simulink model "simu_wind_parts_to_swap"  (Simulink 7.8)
settings: Solver=ode45  StartTime=0.0  StopTime=10.0  RelTol=1e-3
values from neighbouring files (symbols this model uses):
  a = 14.2e-3/2    (= 0.0071)    [hybrid_wind.m]    (also in measurements.m)
  an = modal_coeff(:,1)    [hybrid_wind.m]
  c = 344    [hybrid_wind.m]    (also in measurements.m)
  fs = 1/Ts    (= 40000)    [hybrid_wind.m]    (also in measurements.m)
  mu_s = 0.8    [bowed_string_hyperbolic.m]
  PM = 50    [bowed_string_hyperbolic.m]    (also in lip_reed.m = 20; single_reed.m = 100)
  Qn = modal_coeff(:,3)    [hybrid_wind.m]
  rho = 1.204    [hybrid_wind.m]    (also in measurements.m)
  St = a^2 *pi    (= 0.000158367685667)    [hybrid_wind.m]    (also in measurements.m)
  Ts = 25e-6    (= 2.5e-05)    [hybrid_wind.m]    (also in measurements.m)
  wn = modal_coeff(:,2)    [hybrid_wind.m]
  wr_vect = [timevect_sigs'  wr_start+ (sawtooth(timevect_sigs/5*2*pi)+1)'/2*(wr_stop-wr_start) ]    [lip_reed.m]
undefined symbols (not defined in the file or in its folder): Bl, cell2mat, d1, d2, dL, He_d, Lt, Mms, modal_coeff, n1, Qts, Re, Sd, w_rms, wLS, ws, Zcstring, zetaLS
libraries: fl_lib x7, simulink x5, nesl_utility x4

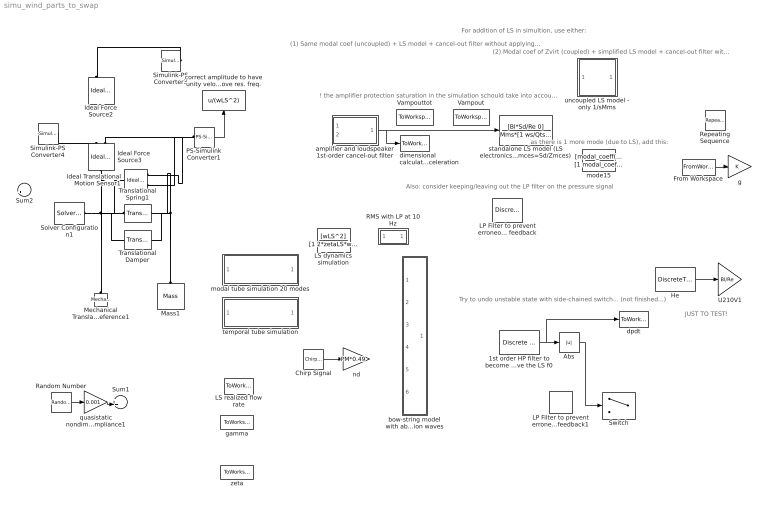
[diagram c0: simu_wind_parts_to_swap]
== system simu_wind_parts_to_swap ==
  note: For addition of LS in simultion, use either:
  note: (1) Same modal coef (uncoupled) + LS model + cancel-out filter without applying the FB
  note: (2) Modal coef of Zvirt (coupled) + simplified LS model + cancel-out filter with applying the FB
  note: as there is 1 more mode (due to LS), add this:
  note: Also: consider keeping/leaving out the LP filter on the pressure signal
  note: Try to undo unstable state with side-chained switch... (not finished...)
  note: ! the amplifier protection saturation in the simulation schould take into account the uncoupling feedback signal...
  note: JUST TO TEST!
  1st order HP filter to become a flat  amp and 0 phase flow rate response above the LS f0 : simulink/Discrete/Discrete Derivative  gainval=1.0  ICPrevScaledInput=0.0  InputProcessing=Inherited  OutMin=[]  OutMax=[]  OutDataType=fixdt(1, 16)  OutScaling=2^-10  DoSatur=off
  Abs : Abs
  Chirp Signal : simulink/Sources/Chirp Signal  f1=0.1  T=5  f2=1000
  From Workspace : FromWorkspace  VariableName=sample  SampleTime=0
  He : DiscreteTransferFcn  Numerator=cell2mat(He_d.num)  Denominator=cell2mat(He_d.den)  SampleTime=Ts
  Ideal Force Source2 : fl_lib/Mechanical/Mechanical Sources/Ideal Force Source  v_Log=off  f_Log=off  LocalVarNames=|v|f  LocalVarDescs=|v|f  LocalVarLogging=[0 0]
  Ideal Force Source3 : fl_lib/Mechanical/Mechanical Sources/Ideal Force Source  v_Log=off  f_Log=off  LocalVarNames=|v|f  LocalVarDescs=|v|f  LocalVarLogging=[0 0]
  Ideal Translational Motion Sensor1 : fl_lib/Mechanical/Mechanical Sensors/Ideal Translational Motion Sensor  offset=0 m  v_Log=off  f_Log=off  x_Log=off  LocalVarNames=|v|f|x  LocalVarDescs=|v|f|x  LocalVarLogging=[0 0 0]
  LP Filter to prevent erroneous high freq feedback : DiscreteFilter  Numerator=HdLP.ScaleValues(1)*HdLP.sosMatrix(1:end/2)  Denominator=HdLP.ScaleValues(2)*HdLP.sosMatrix(1+end/2:end)  SampleTime=Ts
  LP Filter to prevent erroneous high freq feedback1 : DiscreteFilter  Numerator=HdLP.ScaleValues(1)*HdLP.sosMatrix(1:end/2)  Denominator=HdLP.ScaleValues(2)*HdLP.sosMatrix(1+end/2:end)  SampleTime=Ts
  LS dynamics simulation : TransferFcn  Numerator=[wLS^2]  Denominator=[1 2*zetaLS*wLS wLS^2]
  LS realized flow rate : ToWorkspace  VariableName=U_LS  SampleTime=-1  SaveFormat=Structure
  Mass1 : fl_lib/Mechanical/Translational Elements/Mass  mass=1/wLS^2 kg  initial_velocity=0 m/s  f_Log=off  LocalVarNames=|f  LocalVarDescs=|f  LocalVarLogging=0
  Mechanical Translational Reference1 : fl_lib/Mechanical/Translational Elements/Mechanical Translational Reference  f_Log=off  LocalVarNames=|f  LocalVarDescs=|f  LocalVarLogging=0
  PS-Simulink Converter1 : nesl_utility/PS-Simulink Converter  PhysicalDomain=network_engine_domain  LeftPortType=input  RightPortType=output  SubClassName=ps_output  Unit=1  AffineConversion=off
  RMS with LP at 10 Hz : Subsystem
  Random Number : RandomNumber  SampleTime=Ts
  Repeating Sequence : simulink/Sources/Repeating Sequence  rep_seq_t=wr_vect(:,1)/30  rep_seq_y=wr_vect(:,2)
  Simulink-PS Converter3 : nesl_utility/Simulink-PS Converter  PhysicalDomain=network_engine_domain  LeftPortType=input  RightPortType=output  SubClassName=ps_input  Unit=1  AffineConversion=off  InputFilterTimeConstant=.001  UdotUserProvided=0
  Simulink-PS Converter4 : nesl_utility/Simulink-PS Converter  PhysicalDomain=network_engine_domain  LeftPortType=input  RightPortType=output  SubClassName=ps_input  Unit=1  AffineConversion=off  InputFilterTimeConstant=.001  UdotUserProvided=0
  Solver Configuration1 : nesl_utility/Solver Configuration  PhysicalDomain=network_engine_domain  LeftPortType=input  RightPortType=generic  SubClassName=solver  DoDC=on  ResidualTolerance=1e-9  UseLocalSolver=on  LocalSolverChoice=NE_TRAPEZOIDAL_ADVANCER  LocalSolverSampleTime=1/fs  DoFixedCost=on  MaxNonlinIter=3  MaxModeIter=2  LinearAlgebra=Sparse  Accelerate=off  Profile=off  UseLocalSampling=off  DelaysMemoryBudget=1024
  Sum1 : Sum  Inputs=++|
  Sum2 : Sum  Inputs=|+-
  Switch : Switch  Threshold=50
  Translational Damper : fl_lib/Mechanical/Translational Elements/Translational Damper  D=2*zetaLS/wLS N/(m/s)  f_Log=off  v_Log=off  LocalVarNames=|f|v  LocalVarDescs=|f|v  LocalVarLogging=[0 0]
  Translational Spring1 : fl_lib/Mechanical/Translational Elements/Translational Spring  spr_rate=1 N/m  init_def=0 m  f_Log=off  v_Log=off  x_Log=off  LocalVarNames=|f|v|x  LocalVarDescs=|f|v|x  LocalVarLogging=[0 0 0]
  U210V1 : Gain  Gain=Bl/Re
  Vampout : ToWorkspace  VariableName=Vampout  SampleTime=-1  SaveFormat=Structure
  Vampouttot : ToWorkspace  VariableName=Vampouttot  SampleTime=-1  SaveFormat=Structure
  amplifier and loudspeaker 1st-order cancel-out filter : Subsystem
  bow-string model with absorbed torsion waves : Subsystem
  correct amplitude to have unity velocity above res. freq. : Fcn  Expr=u/(wLS^2)
  dimensional calculated flow acceleration : ToWorkspace  VariableName=A  SampleTime=-1  SaveFormat=Structure
  dpdt : ToWorkspace  VariableName=ddpdt  SampleTime=-1  SaveFormat=Structure
  g : Gain
  gamma : ToWorkspace  VariableName=gamma_vect_simu  SampleTime=-1  SaveFormat=Structure
  modal tube simulation 20 modes : Subsystem
  mode15 : TransferFcn  Numerator=[modal_coeff(15, 1) 0]  Denominator=[1 modal_coeff(15,2)/modal_coeff(15,3) modal_coeff(15,2)^2]
  nd : Gain  Gain=PM*0.49
  quasistatic nondimensional reed compliance1 : Gain  Gain=0.001
  standalone LS model (LS electronics&mechanics Bl*Sd/Re*Ymces=Sd/Zmces) : TransferFcn  Numerator=[Bl*Sd/Re 0]  Denominator=Mms*[1 ws/Qts (ws)^2]
  temporal tube simulation : Subsystem
  uncoupled LS model - only 1/sMms : Subsystem
  zeta : ToWorkspace  VariableName=zeta_vect_simu  SampleTime=-1  SaveFormat=Structure
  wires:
  PS-Simulink Converter1/1 -> correct amplitude to have unity velocity above res. freq./1
  correct amplitude to have unity velocity above res. freq./1 -> ?
  Chirp Signal/1 -> nd/1
  1st order HP filter to become a flat  amp and 0 phase flow rate response above the LS f0/1 -> Abs/1, dpdt/1
  Abs/1 -> Switch/2
  Random Number/1 -> quasistatic nondimensional reed compliance1/1
  ? -> Sum1/1  "p_nd"
  quasistatic nondimensional reed compliance1/1 -> Sum1/2
  amplifier and loudspeaker 1st-order cancel-out filter/1(V_amp_out) -> dimensional calculated flow acceleration/1, standalone LS model (LS electronics&mechanics Bl*Sd/Re*Ymces=Sd/Zmces)/1
  He/1 -> U210V1/1
  From Workspace/1 -> g/1
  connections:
  Simulink-PS Converter3/RConn1 -- Ideal Force Source2/RConn1
  Solver Configuration1/RConn1 -- Translational Damper/LConn1 -- Mechanical Translational Reference1/LConn1 -- Translational Spring1/LConn1 -- Ideal Translational Motion Sensor1/LConn1 -- Ideal Force Source3/LConn1
  Ideal Force Source3/RConn2 -- Ideal Translational Motion Sensor1/RConn1 -- Translational Spring1/RConn1 -- Translational Damper/RConn1 -- Mass1/LConn1
  Simulink-PS Converter4/RConn1 -- Ideal Force Source3/RConn1
  Ideal Translational Motion Sensor1/RConn3 -- PS-Simulink Converter1/LConn1

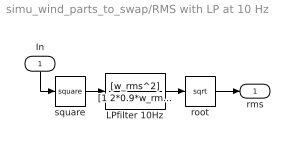
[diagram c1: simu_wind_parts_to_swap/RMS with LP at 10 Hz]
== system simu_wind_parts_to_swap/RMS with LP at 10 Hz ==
  In : Inport
  LPfilter 10Hz : TransferFcn  Numerator=[w_rms^2]  Denominator=[1 2*0.9*w_rms w_rms^2]
  root : Math  Operator=sqrt
  square : Math  Operator=square
  rms : Outport
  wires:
  square/1 -> LPfilter 10Hz/1
  LPfilter 10Hz/1 -> root/1
  In/1 -> square/1
  root/1 -> rms/1

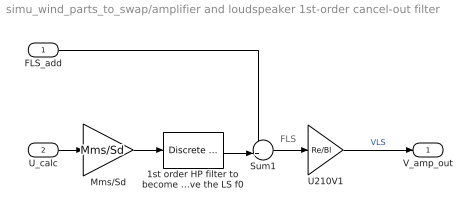
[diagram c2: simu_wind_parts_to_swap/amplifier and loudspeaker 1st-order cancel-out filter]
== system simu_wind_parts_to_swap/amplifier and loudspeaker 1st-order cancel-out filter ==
  note: FLS
  FLS_add : Inport
  U_calc : Inport  Port=2
  1st order HP filter to become a flat  amp and 0 phase flow rate response above the LS f0 : simulink/Discrete/Discrete Derivative  gainval=1.0  ICPrevScaledInput=0.0  InputProcessing=Inherited  OutMin=[]  OutMax=[]  OutDataType=fixdt(1, 16)  OutScaling=2^-10  DoSatur=off
  Mms/Sd : Gain  Gain=Mms/Sd
  Sum1 : Sum  Inputs=-+|
  U210V1 : Gain  Gain=Re/Bl
  V_amp_out : Outport
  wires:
  Sum1/1 -> U210V1/1
  Mms/Sd/1 -> 1st order HP filter to become a flat  amp and 0 phase flow rate response above the LS f0/1
  U210V1/1 -> V_amp_out/1  "VLS"
  U_calc/1 -> Mms/Sd/1
  1st order HP filter to become a flat  amp and 0 phase flow rate response above the LS f0/1 -> Sum1/2
  FLS_add/1 -> Sum1/1

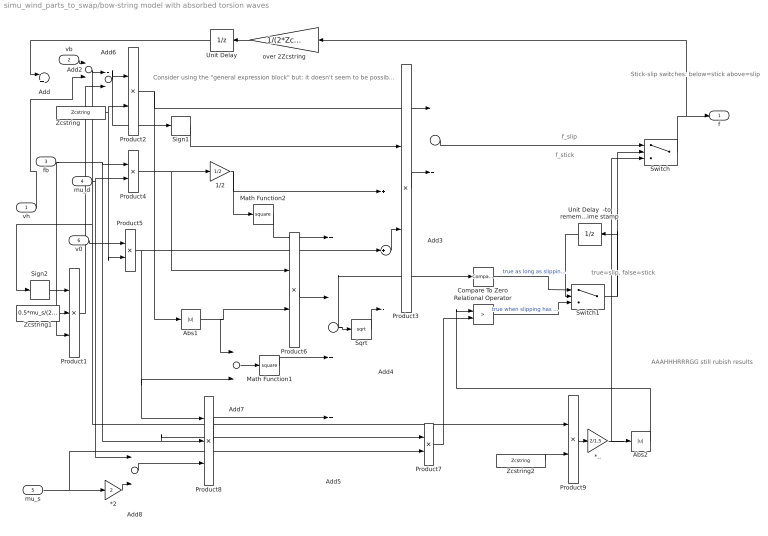
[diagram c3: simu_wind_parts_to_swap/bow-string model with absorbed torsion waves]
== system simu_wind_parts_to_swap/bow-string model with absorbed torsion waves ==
  note: Stick-slip switches: below=stick above=slip
  note: AAAHHHRRRGG still rubish results
  note: true=slip, false=stick
  note: f_stick
  note: f_slip
  note: Consider using the "general expression block" but: it doesn't seem to be possible to make it have more then 1 input! so this way may be more convenient if all parameters are provided as inputs...
  vh : Inport
  vb : Inport  Port=2
  fb : Inport  Port=3
  mu_d : Inport  Port=4
  mu_s : Inport  Port=5
  v0 : Inport  Port=6
  *.. : Gain  Gain=2/1.5
  *2 : Gain  Gain=2
  1/2 : Gain  Gain=1/2
  Abs1 : Abs
  Abs2 : Abs
  Add : Sum  Inputs=-+
  Add2 : Sum  Inputs=+-
  Add3 : Sum
  Add4 : Sum  Inputs=++-
  Add5 : Sum  Inputs=+-++
  Add6 : Sum  Inputs=+-
  Add7 : Sum
  Add8 : Sum  Inputs=+-
  Compare To Zero : simulink/Logic and Bit Operations/Compare To Zero  relop=>  OutDataTypeStr=uint8
  Math Function1 : Math  Operator=square
  Math Function2 : Math  Operator=square
  Product1 : Product  Inputs=3
  Product{2..7,9} (7 alike) : Product
  Product8 : Product  Inputs=3
  Relational Operator : RelationalOperator  Operator=>  OutDataTypeStr=boolean
  Sign1 : Signum
  Sign2 : Signum
  Sqrt : Sqrt
  Switch : Switch  Criteria=u2 > Threshold
  Switch1 : Switch  Criteria=u2 > Threshold
  Unit Delay : UnitDelay  SampleTime=-1
  Unit Delay  -to remember slip/stick state of previous time stamp : UnitDelay  SampleTime=-1
  Zcstring : Constant  Value=Zcstring
  Zcstring1 : Constant  Value=0.5*mu_s/(2*Zcstring)
  Zcstring2 : Constant  Value=Zcstring
  over 2Zcstring : Gain  Gain=1/(2*Zcstring)
  f : Outport
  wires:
  vb/1 -> Add2/1
  Zcstring/1 -> Product2/2, Product5/2
  Product2/1 -> Abs1/1, Add3/1
  Product3/1 -> Add3/2
  fb/1 -> Product4/1, Product8/2, Product7/1, Product1/3
  mu_d/1 -> Product4/2, Add8/1
  Product4/1 -> 1/2/1, Product6/1
  Product5/1 -> Add4/2, Add7/2, Product8/1
  v0/1 -> Product5/1
  Sqrt/1 -> Add4/3
  Sign1/1 -> Product3/1
  Add4/1 -> Product3/2
  Abs1/1 -> Product6/2, Add7/1
  1/2/1 -> Add4/1, Math Function2/1
  Add7/1 -> Math Function1/1
  mu_s/1 -> *2/1, Product7/2
  *2/1 -> Add8/2
  Add8/1 -> Product8/3
  Add5/1 -> Sqrt/1, Compare To Zero/1
  Math Function2/1 -> Add5/1
  Product6/1 -> Add5/2
  Math Function1/1 -> Add5/3
  Product8/1 -> Add5/4
  Add3/1 -> Switch/1
  Switch1/1 -> Unit Delay  -to remember slip/stick state of previous time stamp/1, Switch/2
  Product7/1 -> Relational Operator/2
  Switch/1 -> f/1, over 2Zcstring/1
  Unit Delay  -to remember slip/stick state of previous time stamp/1 -> Switch1/2
  over 2Zcstring/1 -> Unit Delay/1
  Compare To Zero/1 -> Switch1/1  "true as long as slipping is happening"
  Relational Operator/1 -> Switch1/3  "true when slipping has to start"
  Unit Delay/1 -> Add/1
  Zcstring1/1 -> Product1/2
  Sign2/1 -> Product1/1
  Zcstring2/1 -> Product9/2
  Add2/1 -> Add6/1, Sign2/1, Product9/1
  Add6/1 -> Product2/1, Sign1/1
  Product1/1 -> Add6/2
  Product9/1 -> *../1
  Abs2/1 -> Relational Operator/1
  *../1 -> Abs2/1, Switch/3
  vh/1 -> Add2/2

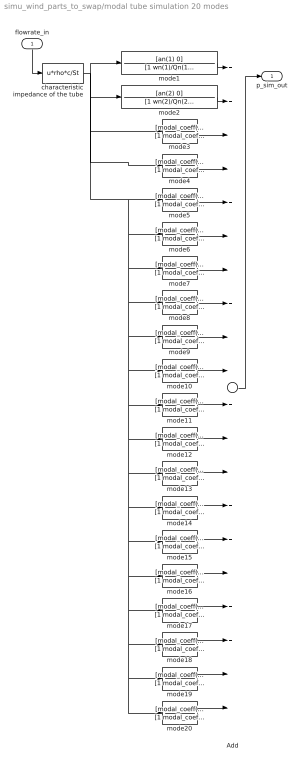
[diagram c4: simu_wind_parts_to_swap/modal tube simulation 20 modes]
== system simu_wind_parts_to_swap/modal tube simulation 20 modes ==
  flowrate_in : Inport
  Add : Sum  Inputs=++++++++++++++++++++
  characteristic impedance of the tube : Fcn  Expr=u*rho*c/St
  mode1 : TransferFcn  Numerator=[an(1) 0]  Denominator=[1 wn(1)/Qn(1) wn(1)^2]
  mode10 : TransferFcn  Numerator=[modal_coeff(10, 1) 0]  Denominator=[1 modal_coeff(10,2)/modal_coeff(10,3) modal_coeff(10,2)^2]
  mode11 : TransferFcn  Numerator=[modal_coeff(11, 1) 0]  Denominator=[1 modal_coeff(11,2)/modal_coeff(11,3) modal_coeff(11,2)^2]
  mode12 : TransferFcn  Numerator=[modal_coeff(12, 1) 0]  Denominator=[1 modal_coeff(12,2)/modal_coeff(12,3) modal_coeff(12,2)^2]
  mode13 : TransferFcn  Numerator=[modal_coeff(13, 1) 0]  Denominator=[1 modal_coeff(13,2)/modal_coeff(13,3) modal_coeff(13,2)^2]
  mode14 : TransferFcn  Numerator=[modal_coeff(14, 1) 0]  Denominator=[1 modal_coeff(14,2)/modal_coeff(14,3) modal_coeff(14,2)^2]
  mode15 : TransferFcn  Numerator=[modal_coeff(15, 1) 0]  Denominator=[1 modal_coeff(15,2)/modal_coeff(15,3) modal_coeff(15,2)^2]
  mode16 : TransferFcn  Numerator=[modal_coeff(16, 1) 0]  Denominator=[1 modal_coeff(16,2)/modal_coeff(16,3) modal_coeff(16,2)^2]
  mode17 : TransferFcn  Numerator=[modal_coeff(17, 1) 0]  Denominator=[1 modal_coeff(17,2)/modal_coeff(17,3) modal_coeff(17,2)^2]
  mode18 : TransferFcn  Numerator=[modal_coeff(18, 1) 0]  Denominator=[1 modal_coeff(18,2)/modal_coeff(18,3) modal_coeff(18,2)^2]
  mode19 : TransferFcn  Numerator=[modal_coeff(19, 1) 0]  Denominator=[1 modal_coeff(19,2)/modal_coeff(19,3) modal_coeff(19,2)^2]
  mode2 : TransferFcn  Numerator=[an(2) 0]  Denominator=[1 wn(2)/Qn(2) wn(2)^2]
  mode20 : TransferFcn  Numerator=[modal_coeff(20, 1) 0]  Denominator=[1 modal_coeff(20,2)/modal_coeff(20,3) modal_coeff(20,2)^2]
  mode3 : TransferFcn  Numerator=[modal_coeff(3, 1) 0]  Denominator=[1 modal_coeff(3,2)/modal_coeff(3,3) modal_coeff(3,2)^2]
  mode4 : TransferFcn  Numerator=[modal_coeff(4, 1) 0]  Denominator=[1 modal_coeff(4,2)/modal_coeff(4,3) modal_coeff(4,2)^2]
  mode5 : TransferFcn  Numerator=[modal_coeff(5, 1) 0]  Denominator=[1 modal_coeff(5,2)/modal_coeff(5,3) modal_coeff(5,2)^2]
  mode6 : TransferFcn  Numerator=[modal_coeff(6, 1) 0]  Denominator=[1 modal_coeff(6,2)/modal_coeff(6,3) modal_coeff(6,2)^2]
  mode7 : TransferFcn  Numerator=[modal_coeff(7, 1) 0]  Denominator=[1 modal_coeff(7,2)/modal_coeff(7,3) modal_coeff(7,2)^2]
  mode8 : TransferFcn  Numerator=[modal_coeff(8, 1) 0]  Denominator=[1 modal_coeff(8,2)/modal_coeff(8,3) modal_coeff(8,2)^2]
  mode9 : TransferFcn  Numerator=[modal_coeff(9, 1) 0]  Denominator=[1 modal_coeff(9,2)/modal_coeff(9,3) modal_coeff(9,2)^2]
  p_sim_out : Outport
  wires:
  flowrate_in/1 -> characteristic impedance of the tube/1
  characteristic impedance of the tube/1 -> mode4/1, mode3/1, mode2/1, mode1/1, mode5/1, mode6/1, mode7/1, mode8/1, mode9/1, mode10/1, mode11/1, mode12/1, mode20/1, mode19/1, mode18/1, mode17/1, mode16/1, mode15/1, mode14/1, mode13/1
  mode1/1 -> Add/1
  Add/1 -> p_sim_out/1
  mode2/1 -> Add/2
  mode3/1 -> Add/3
  mode4/1 -> Add/4
  mode5/1 -> Add/5
  mode6/1 -> Add/6
  mode7/1 -> Add/7
  mode8/1 -> Add/8
  mode9/1 -> Add/9
  mode10/1 -> Add/10
  mode11/1 -> Add/11
  mode12/1 -> Add/12
  mode13/1 -> Add/13
  mode14/1 -> Add/14
  mode15/1 -> Add/15
  mode16/1 -> Add/16
  mode17/1 -> Add/17
  mode18/1 -> Add/18
  mode19/1 -> Add/19
  mode20/1 -> Add/20

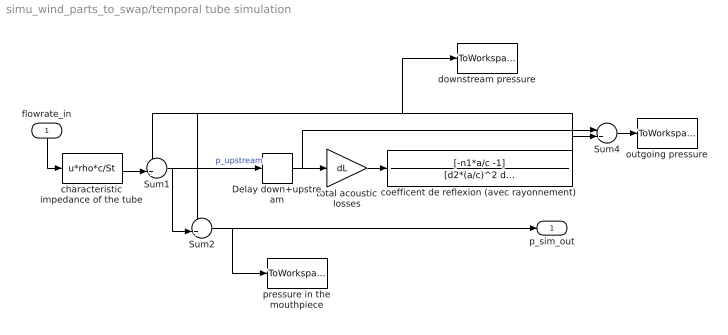
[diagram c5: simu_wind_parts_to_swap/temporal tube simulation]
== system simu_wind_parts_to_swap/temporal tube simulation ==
  flowrate_in : Inport
  Delay down+upstream : TransportDelay  DelayTime=2*Lt/c  BufferSize=512
  Sum1 : Sum  Inputs=++|
  Sum2 : Sum  Inputs=++|
  Sum4 : Sum  Inputs=|+-
  characteristic impedance of the tube : Fcn  Expr=u*rho*c/St
  coefficent de reflexion (avec rayonnement) : TransferFcn  Numerator=[-n1*a/c -1]  Denominator=[d2*(a/c)^2 d1*a/c 1]
  downstream pressure : ToWorkspace  VariableName=p_down  SampleTime=-1  SaveFormat=Structure
  outgoing pressure : ToWorkspace  VariableName=p_out  SampleTime=-1  SaveFormat=Structure
  pressure in the mouthpiece : ToWorkspace  VariableName=p  SampleTime=-1  SaveFormat=Structure
  total acoustic losses : Gain  Gain=dL
  p_sim_out : Outport
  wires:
  characteristic impedance of the tube/1 -> Sum1/2
  Sum1/1 -> Delay down+upstream/1, Sum2/2  "p_upstream"
  Delay down+upstream/1 -> total acoustic losses/1, Sum4/1
  coefficent de reflexion (avec rayonnement)/1 -> Sum1/1, Sum2/1, downstream pressure/1, Sum4/2
  Sum2/1 -> p_sim_out/1, pressure in the mouthpiece/1
  flowrate_in/1 -> characteristic impedance of the tube/1
  total acoustic losses/1 -> coefficent de reflexion (avec rayonnement)/1
  Sum4/1 -> outgoing pressure/1

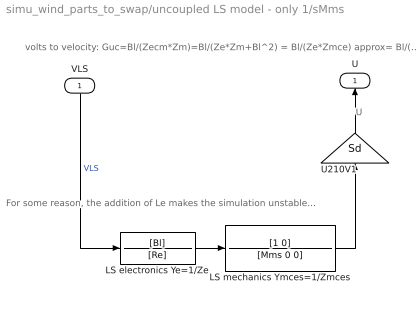
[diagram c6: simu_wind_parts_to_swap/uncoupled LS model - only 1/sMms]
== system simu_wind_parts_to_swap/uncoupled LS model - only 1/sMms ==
  note: U
  note: volts to velocity: Guc=Bl/(Zecm*Zm)=Bl/(Ze*Zm+Bl^2) = Bl/(Ze*Zmce) approx= Bl/(Ze*Zmces) (see "LS-tube interaction measured and calculated.m"...)
  note: For some reason, the addition of Le makes the simulation unstable...
  VLS : Inport
  LS electronics Ye=1/Ze : TransferFcn  Numerator=[Bl]  Denominator=[Re]
  LS mechanics Ymces=1/Zmces : TransferFcn  Numerator=[1 0]  Denominator=[Mms 0 0]
  U210V1 : Gain  Gain=Sd
  U : Outport
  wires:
  LS mechanics Ymces=1/Zmces/1 -> U210V1/1
  VLS/1 -> LS electronics Ye=1/Ze/1  "VLS"
  U210V1/1 -> U/1
  LS electronics Ye=1/Ze/1 -> LS mechanics Ymces=1/Zmces/1
